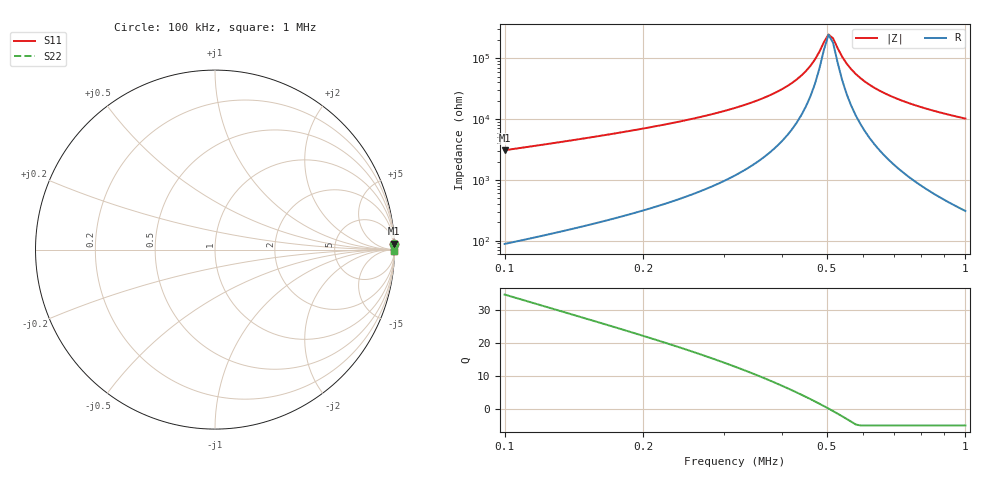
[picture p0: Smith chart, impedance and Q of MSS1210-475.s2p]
# MHz S MA R 50
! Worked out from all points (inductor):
!   102 points, 100 kHz to 1 MHz, reference 50 ohm
!   read as one part in series: L = 4.69 mH near 100 kHz
!   highest Q = 34.8 at 100 kHz (marker M1), where L = 4.89 mH
!   self-resonance near 504.6 kHz
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0.1  0.9985 1.9  0.03251 -86.5  0.03251 -86.5  0.9985 1.9
0.1577683  0.9991 1.1  0.01938 -86.7  0.01938 -86.7  0.9991 1.1
0.2546482  0.9994 0.6  0.009948 -86.2  0.009948 -86.2  0.9994 0.6
0.3424944  0.9995 0.3  0.005388 -84.5  0.005388 -84.5  0.9995 0.3
0.4017542  0.9995 0.2  0.003159 -81.6  0.003159 -81.6  0.9995 0.2
0.430193  0.9996 0.1  0.002237 -78.7  0.002237 -78.7  0.9996 0.1
0.460645  0.9996 0.1  0.001341 -71.7  0.001341 -71.7  0.9996 0.1
0.4712673  0.9996 0.1  0.001053 -66.7  0.001053 -66.7  0.9996 0.1
0.4821346  0.9996 0.0  0.0007793 -58.1  0.0007793 -58.1  0.9996 0.0
0.4932525  0.9996 0.0  0.0005411 -41.3  0.0005411 -41.3  0.9996 0.0
0.5046268  0.9996 0.0  0.0004055 -7.4  0.0004055 -7.4  0.9996 0.0
0.5162633  0.9996 -0.0  0.0004709 32.4  0.0004709 32.4  0.9996 -0.0
0.5281682  0.9996 -0.0  0.0006819 54.7  0.0006819 54.7  0.9996 -0.0
0.5403477  0.9996 -0.0  0.0009458 65.7  0.0009458 65.7  0.9996 -0.0
0.5528079  0.9996 -0.1  0.001229 71.7  0.001229 71.7  0.9996 -0.1
0.5785971  0.9996 -0.1  0.00182 78.0  0.00182 78.0  0.9996 -0.1
0.6195541  0.9996 -0.2  0.002732 82.2  0.002732 82.2  0.9996 -0.2
0.6634103  0.9996 -0.2  0.003664 84.3  0.003664 84.3  0.9996 -0.2
0.7103709  0.9996 -0.3  0.004617 85.5  0.004617 85.5  0.9996 -0.3
0.7781962  0.9997 -0.3  0.005923 86.5  0.005923 86.5  0.9997 -0.3
0.8524974  0.9997 -0.4  0.00728 87.1  0.00728 87.1  0.9997 -0.4
1  0.9997 -0.6  0.009809 87.7  0.009809 87.7  0.9997 -0.6
